// TwinCAT 3 PLC project Novram_FunctionBlocks
// ProgramVersion: 3.1.4023.0
// libraries:
//   Tc2_IoFunctions, * (Beckhoff Automation GmbH)
//   Tc2_Standard, * (Beckhoff Automation GmbH)
//   Tc2_System, * (Beckhoff Automation GmbH)
//   Tc3_Module, * (Beckhoff Automation GmbH)
// project tree:
//   DUTs/ DUT_Novram_Struct.TcDUT
//   / PlcTask.TcTTO
//   POUs/ MAIN.TcPOU
// real-time tasks:
//   TASK PlcTask: cycle T#10ms, priority 20, ADS port 350
// I/O:
//   DEVICE Device 4 (NOV-DP-RAM)

CONFIGURATION Novram_FunctionBlocks
    RESOURCE PLC ON TwinCAT3
        TASK PlcTask(INTERVAL := T#10ms, PRIORITY := 20);
        PROGRAM MAIN WITH PlcTask : MAIN;
    END_RESOURCE
END_CONFIGURATION

// ---- DUTs/DUT_Novram_Struct.TcDUT
TYPE DUT_Novram_Struct :
STRUCT
	s_name: WSTRING;
	i_old: INT;
	s_gender: WSTRING;
	f_height: LREAL;
	f_weight: LREAL;
END_STRUCT
END_TYPE

// ---- POUs/MAIN.TcPOU
PROGRAM MAIN
VAR
	b_read: BOOL;								//触发数据读取
	b_write: BOOL;								//触发数据写入
	
	FB_NovRamReadWriteEx1: FB_NovRamReadWriteEx;
	arr_array: ARRAY[1..100] OF BYTE;			//要写入的数组数据
	arr_array_back: ARRAY[1..100] OF BYTE;		//要读取的数组数据
	
	FB_NovRamReadWriteEx2: FB_NovRamReadWriteEx;
	b_bool: BOOL;
	b_bool_back: BOOL;
	
	FB_NovRamReadWriteEx3: FB_NovRamReadWriteEx;
	i_int: INT;
	i_int_back: INT;
	
	FB_NovRamReadWriteEx4: FB_NovRamReadWriteEx;
	f_real: REAL;
	f_real_back: REAL;
	
	FB_NovRamReadWriteEx5: FB_NovRamReadWriteEx;
	ST_Novram: DUT_Novram_Struct;
	ST_Novram_back: DUT_Novram_Struct;
END_VAR

(*数组变量保持*)
FB_NovRamReadWriteEx1(
	nDevId:= 4,                 	//Novram设备的ID 
	bRead:= b_read, 				//读取Novram区数据
	bWrite:= b_write, 				//写入Novram区数据
	cbSrcLen:= 100, 				//设置写入的数据长度,需根据变量类型计算
	cbDestLen:= 100, 				//设置读取的数据长度,需根据变量类型计算
	pSrcAddr:= ADR(arr_array), 		//指向要写入NOVRAM数据的数据缓冲区的地址指针
	pDestAddr:= ADR(arr_array_back),	//指向要读取NOVRAM数据的数据缓冲区的地址指针 
	nReadOffs:= 0, 					//从NOVRAM中读取数据的地址偏移量,第一个存储区可以设置为0
	nWriteOffs:= 0, 				//NOVRAM中要写入数据的地址偏移量,第一个存储区可以设置为0
	tTimeOut:= , 					//功能块执行时的超时时间
	bBusy=> , 
	bError=> , 
	nErrId=> , 
	cbRead=> , 						//成功读取的数据字节数
	cbWrite=> );					//成功写入的数据字节数
	
(*布尔型变量保持*)
	FB_NovRamReadWriteEx2(
	nDevId:= 4, 
	bRead:= b_read, 
	bWrite:= b_write, 
	cbSrcLen:= 1, 					//BOOL型占1数据长度
	cbDestLen:= 1, 
	pSrcAddr:= ADR(b_bool), 
	pDestAddr:= ADR(b_bool_back), 
	nReadOffs:= 64, 				//可以根据target browser给出的地址信息，计算出数组类型所占地址空间，下一个功能块的地址偏移在原有基础上增加
	nWriteOffs:= 64,
	tTimeOut:= , 
	bBusy=> , 
	bError=> , 
	nErrId=> , 
	cbRead=> , 
	cbWrite=> );
	
	(*整型变量保持*)
	FB_NovRamReadWriteEx3(
	nDevId:= 4, 
	bRead:= b_read, 
	bWrite:= b_write, 
	cbSrcLen:= 2, 
	cbDestLen:= 2, 
	pSrcAddr:= ADR(i_int), 
	pDestAddr:= ADR(i_int_back), 
	nReadOffs:= 65, 
	nWriteOffs:= 65, 
	tTimeOut:= , 
	bBusy=> , 
	bError=> , 
	nErrId=> , 
	cbRead=> , 
	cbWrite=> );
	
	(*浮点型变量保持*)
	FB_NovRamReadWriteEx4(
	nDevId:= 4, 
	bRead:= b_read, 
	bWrite:= b_write, 
	cbSrcLen:= 4, 
	cbDestLen:= 4, 
	pSrcAddr:= ADR(f_real), 
	pDestAddr:= ADR(f_real_back), 
	nReadOffs:= 67, 
	nWriteOffs:= 67, 
	tTimeOut:= , 
	bBusy=> , 
	bError=> , 
	nErrId=> , 
	cbRead=> , 
	cbWrite=> );
	
	(*结构体变量保持*)
	FB_NovRamReadWriteEx5(
	nDevId:= 4, 
	bRead:= b_read, 
	bWrite:= b_write, 
	cbSrcLen:= 344, 
	cbDestLen:= 344, 
	pSrcAddr:= ADR(ST_Novram), 
	pDestAddr:= ADR(ST_Novram_back), 
	nReadOffs:= 71, 
	nWriteOffs:= 71, 
	tTimeOut:= , 
	bBusy=> , 
	bError=> , 
	nErrId=> , 
	cbRead=> , 
	cbWrite=> );

END_PROGRAM
